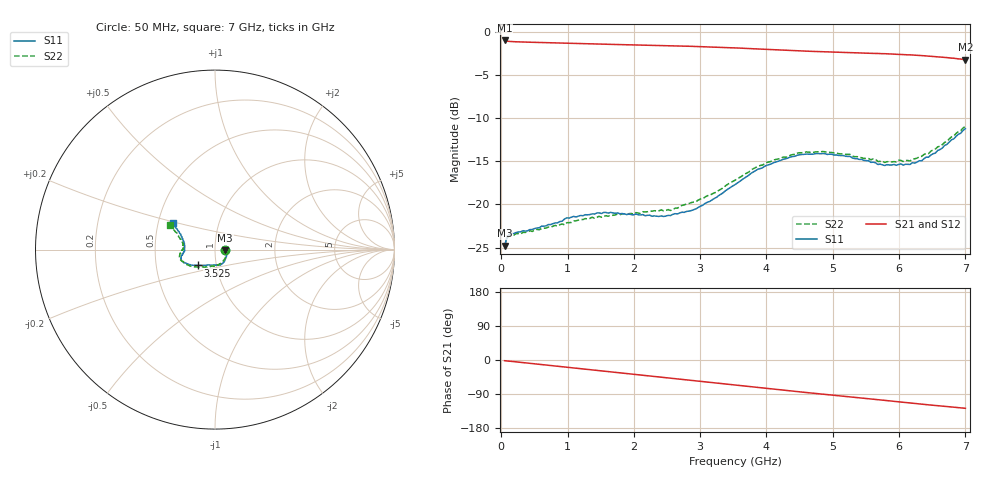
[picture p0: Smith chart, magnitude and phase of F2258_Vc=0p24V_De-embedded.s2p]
! Integrated Device Technology
! Corporate Headquarters
! 6024 Silver Creek Valley Road
! San Jose, CA 95138  USA
! Phone:  1-408-284-8200
! Toll Free:  1-800-223-1366
! Webpage:  http://www.idt.com/
! Timing and RF Division
! 515 Groton Road, Suite 102
! Westford, MA 01886-6024
! Device:  F2258
! Description: Voltage Variable RF Attenuator
! Frequency:  50.0 -  6000.00 MHz
! Package:  3x3 mm Thin QFN Plastic Package: 16 pin
! Ports:  2 RF, 2 DC
!  Pin  1  = NC
!  Pin  2  = NC
!  Pin  3  = RF2  = Port 2
!  Pin  4  = GND
!  Pin  5  = Vdd
!  Pin  6  = NC
!  Pin  7  = VCTRL
!  Pin  8  = NC
!  Pin  9  = GND
!  Pin 10  = RF1  = Port 1
!  Pin 11  = NC
!  Pin 12  = NC
!  Pin 13  = NC
!  Pin 14  = NC
!  Pin 15  = NC
!  Pin 16  = NC
! Vcntrl:  0.240 Volts
! Vdd:  +3.300 Volts
! Current:  1.079 mA
! Data:  The device was measured on a the F2258 evaluation board which has
!  individual transmission lines to the RF pins.  Data was collected
!  using a calibrated network analyzer.  The evaluation board was
!  de-embedded using a TRL calibration technique.
!  The reference plane is the edge of the package pin.
! Misc:  SN 10
!  Action Tracker AT0285
! Date Measured:  2014-12-10
! Date:  2016-01-13  MJV
! Note:
!  Integrated Device Technology supplies this data as a sample of measured
!  data at the package pin for this product.  Your particular data for this
!  product may vary.
!  Data was taken at 25 degrees C.
!  Integrated Device Technology reserves the right to change this data at anytime.
!Freq_(GHz)  S11M_(dB)  S11P_(deg)  S21M_(dB)  S21P_(deg)  S12M_(dB)  S12P_(deg)  S22M_(dB)  S22P_(deg)
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# GHz S dB R 50
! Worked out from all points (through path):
!   201 points, 50 MHz to 7 GHz, reference 50 ohm
!   highest |S21| = -0.96 dB at 50 MHz (marker M1); lowest = -3.2 dB at 7 GHz (marker M2)
!   group delay of S21, straight-line fit = 50.5 ps
!   lowest |S11| = -24.8 dB at 50 MHz (marker M3), VSWR 1.12, Z = 56.1 - j0.391 ohm
!   |S11| at or under -10 dB: start of sweep to end of sweep
!   |S22| runs from -24.8 to -10.9 dB; largest |S21 - S12| = 0.00038
!   S11 on the Smith chart (normalised r, x): 50 MHz: 1.12, -0.01; 3.525 GHz: 0.81, -0.15; 7 GHz: 0.60, +0.19
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0.05  -24.80 -3.5  -0.96 -1.9  -0.96 -1.9  -24.84 -3.0
0.08475  -23.83 -5.9  -1.04 -2.5  -1.04 -2.4  -23.90 -5.4
0.15425  -23.34 -9.2  -1.09 -3.6  -1.09 -3.6  -23.52 -9.4
0.71025  -22.33 -37.0  -1.22 -14.1  -1.22 -14.1  -22.62 -38.5
0.98825  -21.56 -50.8  -1.28 -19.3  -1.28 -19.3  -22.12 -54.6
1.2315  -21.31 -59.1  -1.33 -23.8  -1.33 -23.8  -21.75 -63.5
1.6485  -20.91 -70.8  -1.41 -31.4  -1.41 -31.4  -21.26 -76.5
2.37825  -21.39 -92.1  -1.54 -44.8  -1.54 -44.8  -20.73 -94.2
2.552  -21.29 -98.1  -1.57 -48.0  -1.57 -48.0  -20.70 -99.5
2.93425  -20.53 -114.8  -1.66 -55.1  -1.66 -55.1  -19.70 -112.9
3.247  -19.17 -127.2  -1.74 -61.0  -1.74 -61.0  -18.56 -125.0
3.525  -17.70 -137.5  -1.82 -66.2  -1.82 -66.2  -17.19 -135.5
4.0115  -15.44 -151.2  -2.00 -75.2  -2.00 -75.2  -15.11 -150.9
4.46325  -14.29 -159.6  -2.16 -83.4  -2.17 -83.4  -14.06 -162.0
4.7065  -14.15 -162.9  -2.23 -87.7  -2.24 -87.7  -13.95 -166.3
5.2625  -14.43 -169.8  -2.39 -97.4  -2.39 -97.4  -14.20 -174.3
5.6795  -15.36 -176.6  -2.47 -104.6  -2.47 -104.6  -15.01 -179.7
5.85325  -15.42 179.2  -2.53 -107.8  -2.53 -107.8  -15.04 175.7
6.166  -15.35 171.4  -2.63 -113.4  -2.64 -113.4  -14.95 169.8
6.33975  -14.94 165.1  -2.72 -116.5  -2.72 -116.5  -14.41 165.4
6.722  -13.02 153.4  -2.95 -123.1  -2.95 -123.1  -12.70 156.4
7  -11.21 148.0  -3.19 -127.4  -3.20 -127.4  -10.91 151.5
